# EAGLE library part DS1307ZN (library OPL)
34X8 serial Real-Time Clock
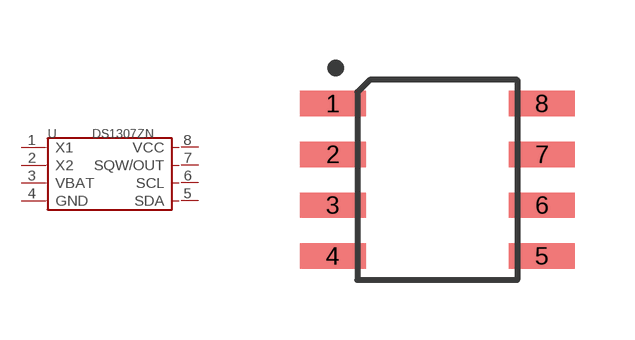
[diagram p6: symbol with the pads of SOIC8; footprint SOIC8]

Designator prefix U

## DS1307ZN-1900100P1  [SOIC8]
1  X1
2  X2
3  VBAT
4  GND
5  SDA
6  SCL
7  SQW/OUT
8  VCC

## Footprint SOIC8 (pad centres in mm)
Small Outline Package
smd 1.651 x 0.635: 1 -2.616,1.905; 2 -2.616,0.635; 3 -2.616,-0.635; 4 -2.616,-1.905; 5 2.616,-1.905; 6 2.616,-0.635; 7 2.616,0.635; 8 2.616,1.905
